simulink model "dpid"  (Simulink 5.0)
settings: Solver=ode4  SolverMode=SingleTasking  StartTime=0.0  StopTime=99.9  FixedStep=.1  RelTol=1e-3  AbsTol=1e-6
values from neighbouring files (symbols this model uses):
  q0 = P+q2    [DPIDrc_S.m]    (also in PID01.m; ab2pq.m = 1.0/sum(B))
  q1 = -P+P*(h/I)-2*q2    [DPIDrc_S.m]    (also in PID01.m)
  q2 = P*(D/h)    [DPIDrc_S.m]    (also in PID01.m)

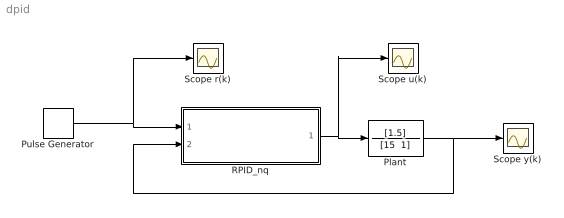
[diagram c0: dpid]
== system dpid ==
  Plant : TransferFcn  Numerator=[1.5]  Denominator="[15  1]"
  Pulse Generator : DiscretePulseGenerator  PulseType=Time based  Period=50  PulseWidth=50
  RPID_nq : Subsystem  mask( PID ){P=.1, I=1.5, D=2, h=.1}
      mask prompts: P "P :"; I "I [s]:"; D "D [s]:"; h "h [s]:"
      mask help: PID: P, I, D - ; h - ;
      mask init:
      | %  Documentation
      |  P=@1;I=@2;D=@3;h=@4;
      | [q0,q1,q2]=pid01(P,I,D,h);
  Scope r(k) : Scope
  Scope u(k) : Scope
  Scope y(k) : Scope
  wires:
  RPID_nq/1(Out1) -> Plant/1, Scope u(k)/1
  Pulse Generator/1 -> RPID_nq/1(In1), Scope r(k)/1
  Plant/1 -> Scope y(k)/1, RPID_nq/2(In2)

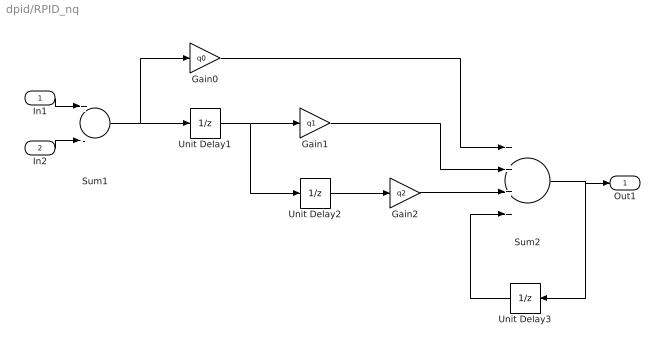
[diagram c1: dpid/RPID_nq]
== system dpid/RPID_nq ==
  In1 : Inport
  In2 : Inport  Port=2
  Gain0 : Gain  Description=GAIN 0  Gain=q0
  Gain1 : Gain  Description=Gain 1  Gain=q1
  Gain2 : Gain  Gain=q2
  Sum1 : Sum  Inputs=+-
  Sum2 : Sum  Inputs=++++
  Unit Delay1 : UnitDelay  Description=Gain 0
  Unit Delay2 : UnitDelay  Description=Gain 1
  Unit Delay3 : UnitDelay  Orientation=left
  Out1 : Outport  InitialOutput=0
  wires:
  Sum1/1 -> Unit Delay1/1, Gain0/1
  Gain0/1 -> Sum2/1
  Unit Delay1/1 -> Gain1/1, Unit Delay2/1
  Unit Delay2/1 -> Gain2/1
  Gain1/1 -> Sum2/2
  Gain2/1 -> Sum2/3
  Sum2/1 -> Unit Delay3/1, Out1/1
  Unit Delay3/1 -> Sum2/4
  In1/1 -> Sum1/1
  In2/1 -> Sum1/2
